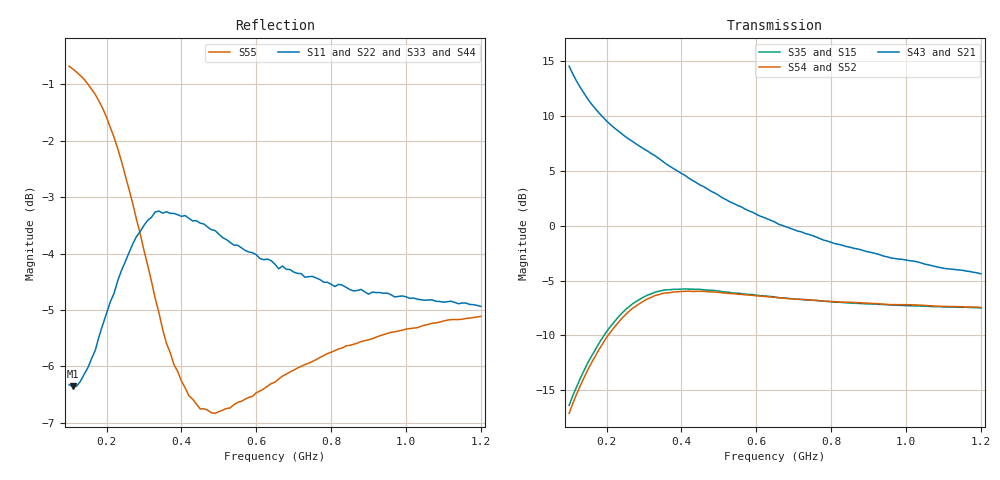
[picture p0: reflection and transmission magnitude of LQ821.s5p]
! SCATTERING PARAMETERS :
!  POLYFET RF DEVICES
!  LQ821 (EACH SIDE)
!  S PARAMETERS
!  VDS=12.5V, IDQ=100mA
!AWR Design Environment (2053) Wed Feb 04 15:20:46 2004
!freq-unit  param-type  data-format  keyword  impedance-ohms
# MHz  S  MA  R  50
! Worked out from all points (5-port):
!   111 points, 100 MHz to 1.2 GHz, reference 50 ohm
!   strongest paths, dB at 100 MHz, 370 MHz, 650 MHz, 930 MHz, 1.2 GHz:
!     S43: 14.6, 5.4, 0.3, -2.6, -4.4
!     S21: 14.6, 5.4, 0.3, -2.6, -4.4
!     S54: -17.1, -6.1, -6.5, -7.1, -7.4
!     S52: -17.1, -6.1, -6.5, -7.1, -7.4
!     S35: -16.4, -5.8, -6.5, -7.2, -7.5
!     S15: -16.4, -5.8, -6.5, -7.2, -7.5
!   lowest |S11| = -6.4 dB at 110 MHz (marker M1), VSWR 2.85, Z = 46.6 - j52.9 ohm
!   |S11| at or under -10 dB: nowhere
